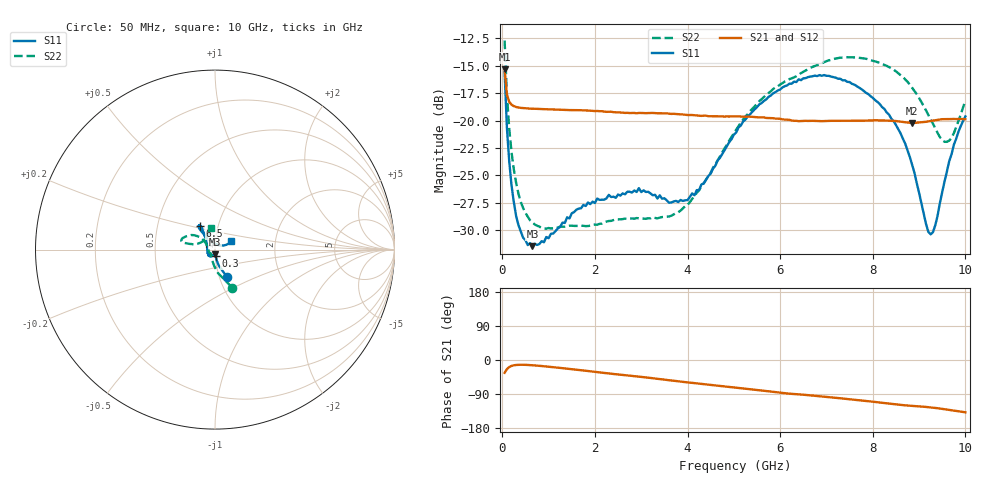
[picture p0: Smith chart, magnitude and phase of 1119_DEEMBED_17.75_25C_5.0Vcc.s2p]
!Hittite Microwave Corp.
!Digital Attenuator/PhaseShifter Rev 1.4.0
!Filename: C:\DATA\DATA\1119_DEEMBED_17.75_25C_5.0Vcc.s2p
!VNA ID: Agilent Technologies,N5224A,MY51441122,A.10.45.03
!Device type:
!2 Port Calibration.
!Temp(C): 25
!Lot Number:
!Serial Number:
!Operator:
!Misc:
!Attenuator:  17.750
# GHZ S DB R 50.0
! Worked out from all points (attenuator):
!   200 points, 50 MHz to 10 GHz, reference 50 ohm
!   highest |S21| = -15.31 dB at 50 MHz (marker M1); lowest = -20.2 dB at 8.85 GHz (marker M2)
!   lowest |S11| = -31.5 dB at 650 MHz (marker M3), VSWR 1.05, Z = 49.8 - j2.66 ohm
!   |S11| at or under -10 dB: start of sweep to end of sweep
!   |S22| runs from -29.9 to -12.7 dB; largest |S21 - S12| = 0.00029
!   S11 on the Smith chart (normalised r, x): 50 MHz: 1.09, -0.34; 300 MHz: 1.00, -0.07; 6.5 GHz: 0.82, +0.22; 10 GHz: 1.20, +0.12
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0.05  -15.55 -66.3  -15.31 -33.8  -15.31 -33.9  -12.68 -65.5
0.1  -20.69 -76.4  -17.64 -24.0  -17.64 -24.0  -17.62 -82.8
0.15  -23.74 -80.4  -18.29 -18.5  -18.29 -18.5  -20.75 -92.5
0.3  -28.75 -85.1  -18.76 -13.1  -18.76 -13.1  -25.71 -109.5
0.45  -30.70 -87.1  -18.85 -12.6  -18.86 -12.6  -27.99 -120.0
0.65  -31.47 -93.3  -18.91 -13.9  -18.91 -13.9  -29.30 -128.7
1.75  -27.71 -118.7  -19.07 -27.7  -19.07 -27.7  -29.61 -138.5
2.95  -26.17 -136.1  -19.30 -43.9  -19.31 -43.9  -28.93 -157.5
3.4  -26.83 -155.3  -19.33 -50.3  -19.34 -50.4  -28.86 -170.8
3.6  -27.50 -166.6  -19.37 -53.4  -19.38 -53.5  -28.76 -178.3
4.15  -26.82 160.7  -19.51 -61.1  -19.52 -61.2  -26.91 158.7
5.05  -21.09 128.3  -19.62 -72.8  -19.64 -72.8  -20.83 140.3
5.75  -17.83 122.7  -19.77 -82.7  -19.78 -82.8  -17.48 144.4
6.5  -16.14 122.3  -20.04 -91.6  -20.05 -91.6  -15.54 152.6
6.7  -15.96 123.1  -20.02 -94.0  -20.03 -94.0  -15.09 154.9
7.5  -16.48 126.5  -20.01 -103.7  -20.02 -103.7  -14.22 164.0
8.35  -19.45 125.9  -20.01 -115.0  -20.01 -115.0  -15.11 167.6
8.85  -24.04 118.7  -20.21 -121.0  -20.21 -121.0  -17.00 167.1
9.25  -30.39 70.5  -20.04 -125.1  -20.06 -125.1  -19.90 161.2
9.35  -29.55 47.5  -19.97 -126.5  -19.99 -126.5  -20.72 156.1
9.65  -23.72 23.5  -19.86 -131.6  -19.87 -131.6  -21.83 126.7
10  -19.62 28.4  -19.87 -138.0  -19.88 -138.0  -18.16 99.5
